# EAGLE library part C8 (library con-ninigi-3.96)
NINIGI
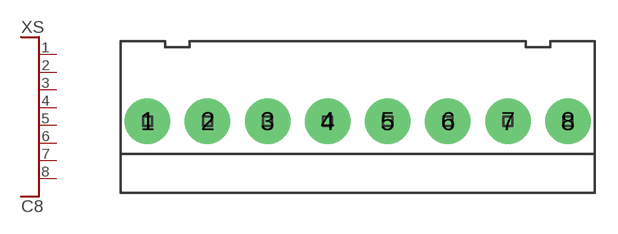
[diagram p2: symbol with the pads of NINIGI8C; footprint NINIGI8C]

Designator prefix XS

## C8  [NINIGI8C]
1  P$1
2  P$2
3  P$3
4  P$4
5  P$5
6  P$6
7  P$7
8  P$8

## Footprint NINIGI8C (pad centres in mm)
drill 1.6 pad 3: 1 -13.86,0; 2 -9.9,0; 3 -5.94,0; 4 -1.98,0; 5 1.98,0; 6 5.94,0; 7 9.9,0; 8 13.86,0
